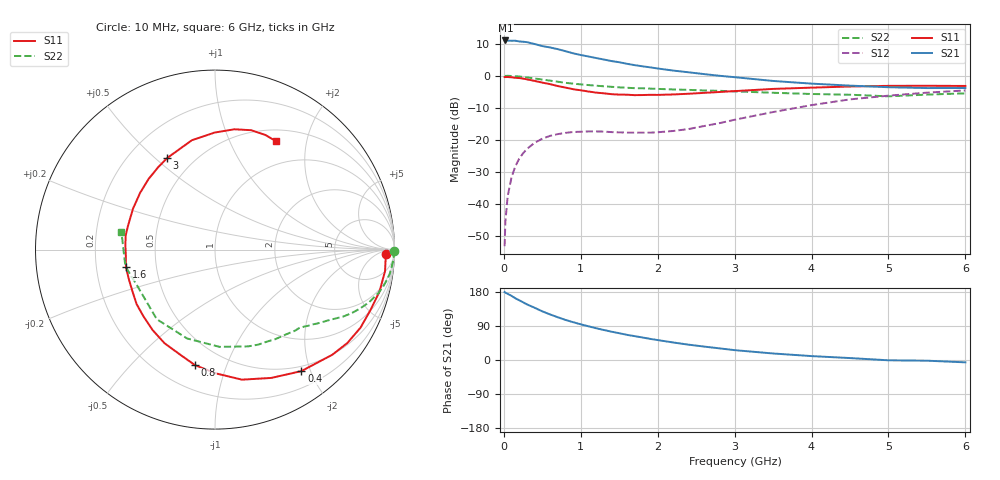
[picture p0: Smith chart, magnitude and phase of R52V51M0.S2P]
! SIEMENS Small Signal Semiconductors
! BFR183
! Si NPN RF Bipolar Junction Transistor in SOT23
! VCE = 2.5 V  IC = 1 mA
! Common Emitter S-Parameters:  May  1996
# GHz  S  MA  R  50
!  f  S11  S21  S12  S22
! GHz  MAG  ANG  MAG  ANG  MAG  ANG  MAG  ANG
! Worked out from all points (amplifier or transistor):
!   36 points, 10 MHz to 6 GHz, reference 50 ohm
!   highest |S21| = 11.0 dB at 20 MHz (marker M1)
!   |S21| within 3 dB of that: start of sweep to 746.7 MHz
!   unconditionally stable (mu >= 1): 1.637 GHz to 2.956 GHz
!   at 250 MHz: K = 0.15, MSG = 17.4 dB, |S12| = -24.2 dB
!   at 1.4 GHz: K = 0.86, MSG = 11.1 dB, |S12| = -17.6 dB
!   at 6 GHz: K = 0.96, MSG = 0.4 dB, |S12| = -4.6 dB
!   S11 on the Smith chart (normalised r, x): 10 MHz: 34, -17; 400 MHz: 0.43, -1.86; 800 MHz: 0.35, -0.78; 1.6 GHz: 0.33, -0.09; 3 GHz: 0.36, +0.55; 6 GHz: 0.65, +1.50
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0.01  0.9542 -1.4  3.481 179.3  0.0022 88.9  0.9989 -0.5
0.02  0.952 -2.7  3.548 177.7  0.0053 87.6  0.9916 -1.0
0.05  0.955 -7.2  3.53 174.6  0.0132 85.6  0.9974 -2.7
0.1  0.9457 -14.4  3.506 169.3  0.0262 82.1  0.9898 -5.2
0.15  0.9289 -21.5  3.512 162.8  0.0387 76.7  0.9828 -7.9
0.3  0.8776 -41.9  3.34 146.8  0.0723 65.5  0.9421 -14.9
0.4  0.8306 -54.6  3.122 137.9  0.09 58.5  0.9071 -18.9
0.5  0.7808 -66.3  2.898 128.4  0.1042 52.4  0.8724 -22.1
0.6  0.74 -78.3  2.761 120.3  0.1155 47.4  0.839 -25.0
0.7  0.6909 -89.2  2.599 112.9  0.1229 42.9  0.8068 -27.5
0.8  0.6539 -99.7  2.416 105.9  0.1285 39.0  0.7757 -29.6
0.9  0.6165 -108.4  2.237 99.8  0.1325 36.3  0.7523 -31.3
1.1  0.5673 -127.8  1.995 88.9  0.1354 32.0  0.7152 -34.7
1.3  0.532 -145.2  1.79 79.2  0.1346 29.9  0.6846 -37.5
1.6  0.5058 -168.8  1.536 66.4  0.1298 31.1  0.6491 -41.8
1.9  0.5039 171.1  1.352 55.8  0.1296 36.4  0.6302 -46.7
2.2  0.5105 153.6  1.204 46.3  0.1375 44.0  0.6112 -51.8
3  0.5756 117.6  0.949 26.0  0.2059 56.4  0.5702 -71.0
3.5  0.623 101.9  0.829 17.2  0.2715 55.1  0.5425 -87.3
4.5  0.6791 80.8  0.701 5.1  0.4278 42.0  0.5056 -129.9
5.5  0.6976 66.2  0.642 -1.8  0.5446 24.8  0.508 -169.4
6  0.6928 60.8  0.643 -6.2  0.5902 14.7  0.531 169.1
